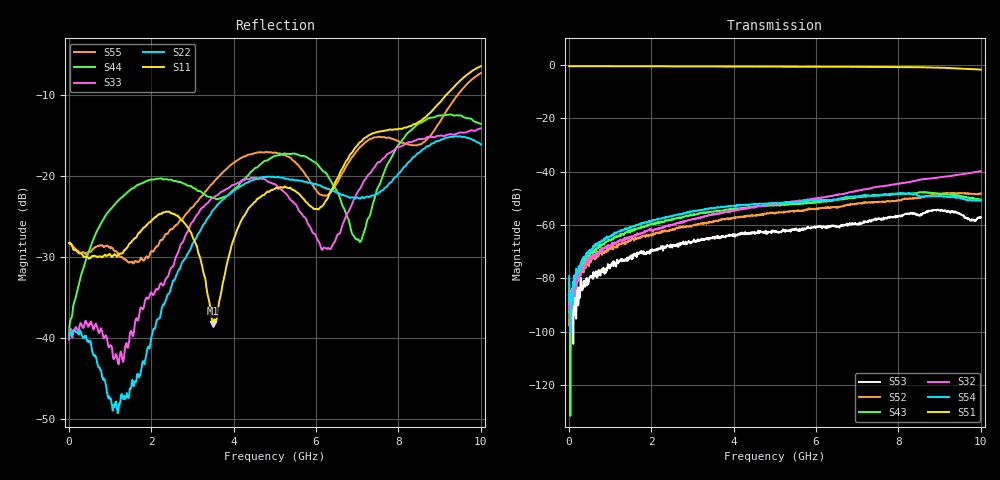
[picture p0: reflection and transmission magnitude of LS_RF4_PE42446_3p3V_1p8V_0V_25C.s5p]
! Created Wed Jan 31 17:43:33 2024
# ghz S ma R 50
! 5 Port Network Data from SP1.SP block
! freq  magS11  angS11  magS12  angS12  magS13  angS13  magS14  angS14
!  magS15  angS15
!  magS21  angS21  magS22  angS22  magS23  angS23
!  magS24  angS24  magS25  angS25
!  magS31  angS31  magS32  angS32
!  magS33  angS33  magS34  angS34  magS35  angS35
!  magS41  angS41
!  magS42  angS42  magS43  angS43  magS44  angS44  magS45  angS45
!  magS51  angS51  magS52  angS52  magS53  angS53  magS54  angS54
!  magS55  angS55
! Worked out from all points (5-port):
!   1000 points, 10 MHz to 10 GHz, reference 50 ohm
!   strongest paths, dB at 10 MHz, 2.51 GHz, 5.01 GHz, 7.51 GHz, 10 GHz:
!     S51: -0.5, -0.6, -0.7, -0.8, -1.8
!     S54: -79.1, -56.6, -51.8, -48.9, -50.8
!     S32: -91.6, -59.8, -52.2, -45.6, -39.8
!     S43: -92.5, -57.8, -52.5, -48.7, -50.6
!     S52: -81.4, -61.9, -55.7, -51.4, -48.2
!     S53: -81.3, -68.5, -62.3, -57.5, -57.1
!   lowest |S11| = -38.2 dB at 3.5 GHz (marker M1), VSWR 1.02, Z = 48.8 - j0.24 ohm
!   |S11| at or under -10 dB: start of sweep to 9.15 GHz
